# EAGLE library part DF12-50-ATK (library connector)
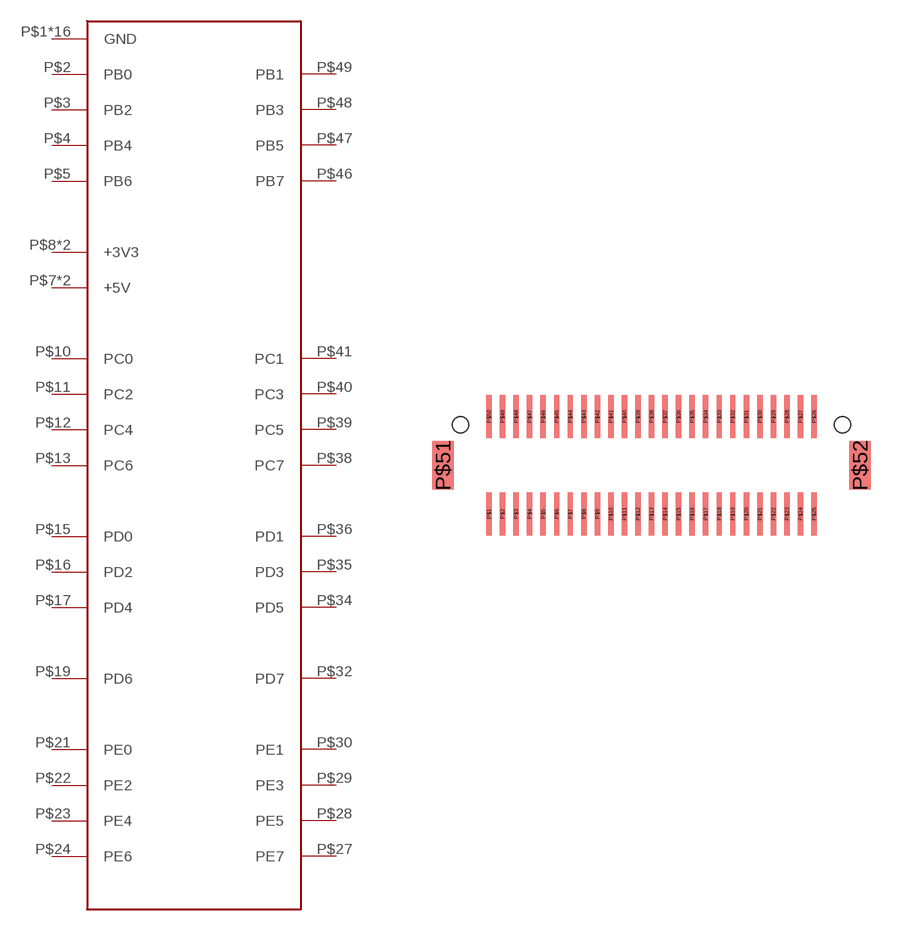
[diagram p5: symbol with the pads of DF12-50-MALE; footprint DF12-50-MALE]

Designator prefix J

## DF12-50-ATK  [DF12-50-MALE]
P$1  GND
P$2  PB0
P$3  PB2
P$4  PB4
P$5  PB6
P$6  GND
P$7  +5V
P$8  +3V3
P$9  GND
P$10  PC0
P$11  PC2
P$12  PC4
P$13  PC6
P$14  GND
P$15  PD0
P$16  PD2
P$17  PD4
P$18  GND
P$19  PD6
P$20  GND
P$21  PE0
P$22  PE2
P$23  PE4
P$24  PE6
P$25  GND
P$26  GND
P$27  PE7
P$28  PE5
P$29  PE3
P$30  PE1
P$31  GND
P$32  PD7
P$33  GND
P$34  PD5
P$35  PD3
P$36  PD1
P$37  GND
P$38  PC7
P$39  PC5
P$40  PC3
P$41  PC1
P$42  GND
P$43  +3V3
P$44  +5V
P$45  GND
P$46  PB7
P$47  PB5
P$48  PB3
P$49  PB1
P$50  GND
P$51  GND
P$52  GND

## Footprint DF12-50-MALE (pad centres in mm)
smd 0.2 x 1.6: P$1 -6,-1.8; P$2 -5.5,-1.8; P$3 -5,-1.8; P$4 -4.5,-1.8; P$5 -4,-1.8; P$6 -3.5,-1.8; P$7 -3,-1.8; P$8 -2.5,-1.8; P$9 -2,-1.8; P$10 -1.5,-1.8; P$11 -1,-1.8; P$12 -0.5,-1.8; P$13 0,-1.8; P$14 0.5,-1.8; P$15 1,-1.8; P$16 1.5,-1.8; P$17 2,-1.8; P$18 2.5,-1.8; P$19 3,-1.8; P$20 3.5,-1.8; P$21 4,-1.8; P$22 4.5,-1.8; P$23 5,-1.8; P$24 5.5,-1.8; P$25 6,-1.8; P$26 6,1.8; P$27 5.5,1.8; P$28 5,1.8; P$29 4.5,1.8; P$30 4,1.8; P$31 3.5,1.8; P$32 3,1.8; P$33 2.5,1.8; P$34 2,1.8; P$35 1.5,1.8; P$36 1,1.8; P$37 0.5,1.8; P$38 0,1.8; P$39 -0.5,1.8; P$40 -1,1.8; P$41 -1.5,1.8; P$42 -2,1.8; P$43 -2.5,1.8; P$44 -3,1.8; P$45 -3.5,1.8; P$46 -4,1.8; P$47 -4.5,1.8; P$48 -5,1.8; P$49 -5.5,1.8; P$50 -6,1.8
smd 0.8 x 1.8: P$51 -7.7,0; P$52 7.7,0
hole 0.6 at -7.05,1.5
hole 0.6 at 7.05,1.5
